//DB986.AWL
// ***************************************************************************


DATA_BLOCK "XC_SEBU_SR"
TITLE = Cross Coupling jobs

AUTHOR: 	SIEMENS
FAMILY: 	SISTARS7
NAME:		XCSEBUSR
VERSION: 	4.02

//$NOW_HOW_PROTECT

//
// Datum		Name			Aktion
// ----------------------------------------------------------------------------
// 19.05.99 	Mahler		Neu

  STRUCT

        SendData		: ARRAY[1..15] of "XC_BUFF_SR_UDT" ;

END_STRUCT ;

BEGIN

END_DATA_BLOCK

